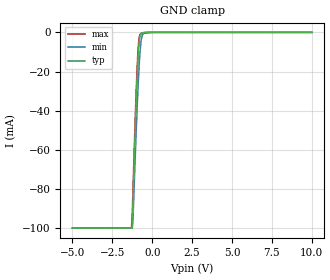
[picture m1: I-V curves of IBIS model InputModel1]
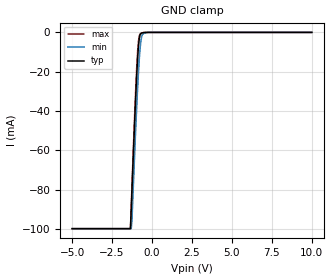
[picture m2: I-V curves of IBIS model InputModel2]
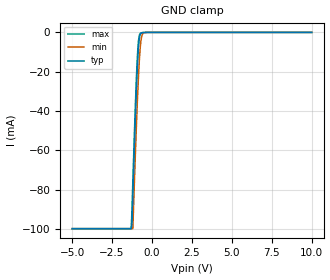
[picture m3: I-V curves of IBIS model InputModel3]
[IBIS Ver]   2.1
[File name]   pa008sa5.ibs   | pa= PSOP, f0008sa= abbr chip name, 5= 5V Vcc
[File Rev]   2.00
[Date]   23-February-96
[Source]   File generated from lab measurements at Intel Corporation
[Notes]   Rev 2.00 All data was replaced by actual measurements
   performed in a lab.
[Disclaimer] INTEL DEVELOPER'S SOFTWARE LICENSE AGREEMENT
| BY USING THIS SOFTWARE, YOU ARE AGREEING TO BE BOUND
| BY THE TERMS OF THIS AGREEMENT.  DO NOT USE THE SOFTWARE
| UNTIL YOU HAVE CAREFULLY READ AND AGREED TO THE FOLLOWING
| TERMS AND CONDITIONS.  IF YOU DO NOT AGREE TO THE TERMS
| OF THIS AGREEMENT, PROMPTLY RETURN THE SOFTWARE PACKAGE
| AND ANY ACCOMPANYING ITEMS.
| IF YOU USE THIS SOFTWARE, YOU WILL BE BOUND BY THE TERMS
| OF THIS AGREEMENT
| LICENSE: Intel Corporation ("Intel") grants you the non-exclusive right
| to use the enclosed software program ("Software").  You will not use,
| copy, modify, rent, sell or transfer the Software or any portion
| thereof, except as provided in this Agreement.
| System OEM Developers may:
| 1.   Copy the Software for support, backup or archival purposes;
| 2.   Install, use, or distribute Intel owned Software in object code
|   only;
| 3.   Modify and/or use Software source code that Intel directly makes
|   available to you as an OEM Developer;
| 4.   Install, use, modify, distribute, and/or make or have made
|   derivatives ("Derivatives") of Intel owned Software under the
|   terms and conditions in this Agreement, ONLY if you are a System
|   OEM Developer and NOT an end-user.
| RESTRICTIONS:
| YOU WILL NOT:
| 1.   Copy the Software, in whole or in part, except as provided for
|   in this Agreement;
| 2.   Decompile or reverse engineer any Software provided in object
|   code format;
| 3.   Distribute any Software or Derivative code to any end-users,
|   unless approved by Intel in a prior writing.
| TRANSFER: You may transfer the Software to another OEM
| Developer if the receiving party agrees to the terms of this
| Agreement at the sole risk of any receiving party.
| OWNERSHIP AND COPYRIGHT OF SOFTWARE:
| Title to the Software and all copies thereof remain with Intel
| or its vendors.  The Software is copyrighted and is protected by
| United States and international copyright laws.  You will not
| remove the copyright notice from the Software.  You agree to
| prevent any unauthorized copying of the Software.
| DERIVATIVE WORK: OEM Developers that make or have made
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[Copyright]   Copyright 1996, Intel Corporation, All Rights Reserved
[Component]   PA28F008SA   | 44-lead PSOP package, 28F008SA
[Manufacturer]  Intel   | Boot Block (tm)
|   | operating in 5V Vcc range
[Package]
|The following values apply for the leadframe.
|Variable   typ   min   max
R_pkg   145.5m   144.0m   147.0m
L_pkg   5.25nH   2.00nH   8.50nH
C_pkg   1.09pF   0.68pF   1.50pF
|*****************************Pin Definitions**********************************
[Pin]   signal_name   model_name   R_pin   L_pin   C_pin
  1   VPP   POWER
  2   RP#   InputModel4
  3   A11   InputModel2
  4   A10   InputModel2
  5   A09   InputModel2
  6   A08   InputModel2
  7   A07   InputModel2
  8   A06   InputModel2
  9   A05   InputModel2
 10   A04   InputModel2
 11   NC   InputModel5
 12   NC   InputModel5
 13   A03   InputModel1
 14   A02   InputModel1
 15   A01   InputModel1
 16   A00   InputModel1
 17   DQ0   InputOutput
 18   DQ1   InputOutput
 19   DQ2   InputOutput
 20   DQ3   InputOutput
 21   GND   GND
 22   GND   GND
 23   VCC   POWER
 24   DQ4   InputOutput
 25   DQ5   InputOutput
 26   DQ6   InputOutput
 27   DQ7   InputOutput
 28   RY/BY#   RYBYOutput
 29   OE#   InputModel3
 30   WE#   InputModel3
 31   NC   InputModel5
 32   NC   InputModel5
 33   NC   InputModel5
 34   NC   InputModel5
 35   A19   InputModel2
 36   A18   InputModel2
 37   A17   InputModel2
 38   A16   InputModel2
 39   A15   InputModel2
 40   A14   InputModel2
 41   A13   InputModel2
 42   A12   InputModel2
 43   CE#   InputModel3
 44   VCC   POWER
|**********************Input Model 5***************************************
[Model]   InputModel5
Model_type   Input
|   For NC pins
Vinl = 0.8V
Vinh = 2.0V
| Variable   typ   min   max
C_comp   5.61p   NA   7.6p
[Voltage Range]   5.0V   4.5V   5.5V
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| Models and submodels in the file (7): InputModel1 (Input), InputModel2 (Input), InputModel3 (Input), InputModel4 (Input), InputModel5 (Input), InputOutput (I/O), RYBYOutput (Output)
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|**************************Input Model 1***************************************
[Model]   InputModel1
Model_type   Input
|   For A[3:0]
Vinl = 0.8V
Vinh = 2.0V
| Variable   typ   min   max
C_comp   5.61p   NA   7.6p
[Voltage Range]   5.0V   4.5V   5.5V
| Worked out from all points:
|   GND clamp passes 1 mA (typ) near -0.72 V on its own axis
[GND_clamp]
|Voltage I(typ)   I(min)   I(max)
-5V       -99.85mA   -99.84mA   -99.85mA
-1.3V     -99.85mA   -99.84mA   -99.85mA
-1.25V    -99.83mA   -99.84mA   -92.56mA
-1.2V     -85.91mA   -94.75mA   -78.96mA
-1.05V    -46.93mA   -60.78mA   -40.45mA
-950mV    -24.37mA   -39.94mA   -18.85mA
-850mV    -8.175mA   -22.06mA   -4.862mA
-800mV    -3.667mA   -14.55mA   -1.917mA
-700mV    -717.5uA   -4.645mA   -522.5uA
-600mV    -274uA     -1.047mA   -226.9uA
0V        0A         0A         0A
10V       0A         0A         0A
[POWER_clamp]
| Input buffer circuits of this product do not intrinsically
| require a [POWER_clamp] definition.  This zero current
| [POWER_clamp] is provided for compatibility with some ibis
| parsers.
|   Voltage  I(typ)   I(min)   I(max)
-5V       0A         0A         0A
-4.75V    0A         0A         0A
9.75V     0A         0A         0A
10V       0A         0A         0A
|**********************Input Model 2************************************
[Model]   InputModel2
Model_type   Input
|   For A[19:4]
Vinl = 0.8V
Vinh = 2.0V
| Variable   typ   min   max
C_comp   5.61p   NA   7.6p
[Voltage Range]   5.0V   4.5V   5.5V
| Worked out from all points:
|   GND clamp passes 1 mA (typ) near -0.73 V on its own axis
[GND_clamp]
|Voltage I(typ)   I(min)   I(max)
-5V       -99.84mA   -99.84mA   -99.84mA
-1.35V    -99.84mA   -99.84mA   -99.84mA
-1.3V     -90.06mA   -99.84mA   -88.39mA
-1.25V    -79.28mA   -94.68mA   -77.04mA
-1.1V     -48.07mA   -64.47mA   -44.59mA
-950mV    -20.49mA   -36.5mA    -16.5mA
-850mV    -7.244mA   -20.62mA   -4.445mA
-750mV    -1.356mA   -8.439mA   -748.5uA
-700mV    -613.5uA   -4.588mA   -433.7uA
-600mV    -217.8uA   -1.014mA   -177.9uA
-250mV    0A         0A         0A
10V       0A         0A         0A
[POWER_clamp]
| Input buffer circuits of this product do not intrinsically
| require a [POWER_clamp] definition.  This zero current
| [POWER_clamp] is provided for compatibility with some ibis
| parsers.
|   Voltage  I(typ)   I(min)   I(max)
-5V       0A         0A         0A
-4.75V    0A         0A         0A
9.75V     0A         0A         0A
10V       0A         0A         0A
|*********************Input Model 3**************************************
[Model]   InputModel3
Model_type   Input
|   For WE#, OE# & CE#
Vinl = 0.8V
Vinh = 2.0V
| Variable   typ   min   max
C_comp   5.61p   NA   7.6p
[Voltage Range]   5.0V   4.5V   5.5V
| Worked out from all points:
|   GND clamp passes 1 mA (typ) near -0.73 V on its own axis
[GND_clamp]
|Voltage I(typ)   I(min)   I(max)
-5V       -99.85mA   -99.84mA   -99.85mA
-1.3V     -99.85mA   -99.84mA   -99.85mA
-1.25V    -96.72mA   -99.84mA   -89.03mA
-1.2V     -83.27mA   -99.84mA   -75.92mA
-1.05V    -45.34mA   -63.96mA   -38.88mA
-950mV    -23.44mA   -41.82mA   -18.03mA
-900mV    -14.49mA   -31.8mA    -10.01mA
-850mV    -7.737mA   -22.92mA   -4.505mA
-750mV    -1.246mA   -8.932mA   -592.5uA
-650mV    -239.3uA   -2.195mA   -180.6uA
-500mV    -36.72uA   -152.6uA   -55.65uA
10V       0A         0A         0A
[POWER_clamp]
| Input buffer circuits of this product do not intrinsically
| require a [POWER_clamp] definition.  This zero current
| [POWER_clamp] is provided for compatibility with some ibis
| parsers.
|   Voltage  I(typ)   I(min)   I(max)
-5V       0A         0A         0A
-4.75V    0A         0A         0A
9.75V     0A         0A         0A
10V       0A         0A         0A
